FUNCTION_BLOCK FB_DO_IED_LD1_MMXU1_PhV_phsA EXTENDS FB_AcsiCommonDataClass
VAR_INPUT
	cVal: FB_AcsiDATypeVector := (fc:=ACSI_FC_MX, TrgOp:=ACSI_TrgOp_dchg OR ACSI_TrgOp_dupd, bLinkResult:=THIS^.AddDataToContainer(ipData:=cVal));
	q: FB_AcsiDATypeQuality := (fc:=ACSI_FC_MX, TrgOp:=ACSI_TrgOp_qchg, bLinkResult:=THIS^.AddDataToContainer(ipData:=q));
	t: FB_AcsiDATypeTimeStamp := (fc:=ACSI_FC_MX, bLinkResult:=THIS^.AddDataToContainer(ipData:=t));
END_VAR
VAR
END_VAR

END_FUNCTION_BLOCK
